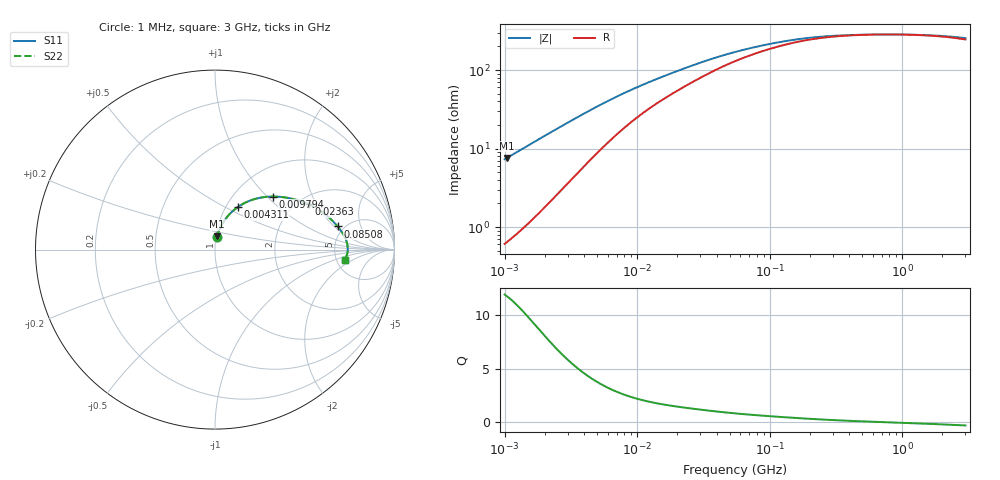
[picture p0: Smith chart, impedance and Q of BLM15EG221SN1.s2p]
! BLM15EG221SN1
# Hz S RI R 50
!Freq.(Hz) S11(Real) S11(Imag) S21(Real) S21(Imag) S12(Real) S12(Imag) S22(Real) S22(Imag)
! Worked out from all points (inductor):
!   401 points, 1 MHz to 3 GHz, reference 50 ohm
!   read as one part in series: L = 1.15 uH near 1.041 MHz
!   highest Q = 11.8 at 1.041 MHz (marker M1), where L = 1.16 uH
!   self-resonance near 825.3 MHz
!   S11 on the Smith chart (normalised r, x): 1 MHz: 1.01, +0.15; 4.311 MHz: 1.14, +0.59; 9.794 MHz: 1.49, +1.09; 23.63 MHz: 2.28, +1.73; 85.08 MHz: 4.41, +2.21; 3 GHz: 5.91, -1.39
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1000000  0.0112 0.0715  0.9888 -0.0715  0.9888 -0.0715  0.0112 0.0715
1040844  0.012 0.0743  0.988 -0.0743  0.988 -0.0743  0.012 0.0743
1553251  0.0235 0.1084  0.9765 -0.1084  0.9765 -0.1084  0.0235 0.1084
2182827  0.0426 0.1465  0.9574 -0.1465  0.9574 -0.1465  0.0426 0.1465
2947212  0.0712 0.1863  0.9288 -0.1863  0.9288 -0.1863  0.0712 0.1863
3823119  0.108 0.2225  0.892 -0.2225  0.892 -0.2225  0.108 0.2225
4310966  0.1293 0.2385  0.8707 -0.2385  0.8707 -0.2385  0.1293 0.2385
5266264  0.1704 0.2623  0.8296 -0.2623  0.8296 -0.2623  0.1704 0.2623
6433254  0.2175 0.2806  0.7825 -0.2806  0.7825 -0.2806  0.2175 0.2806
7858845  0.2681 0.2917  0.7319 -0.2917  0.7319 -0.2917  0.2681 0.2917
9794439  0.3247 0.2956  0.6753 -0.2956  0.6753 -0.2956  0.3247 0.2956
1.461624e7  0.422 0.2848  0.578 -0.2848  0.578 -0.2848  0.422 0.2848
2.362996e7  0.5232 0.2522  0.4768 -0.2522  0.4768 -0.2522  0.5232 0.2522
3.597591e7  0.594 0.2121  0.406 -0.2121  0.406 -0.2121  0.594 0.2121
5.477226e7  0.6456 0.1693  0.3544 -0.1693  0.3544 -0.1693  0.6456 0.1693
8.507507e7  0.6832 0.1291  0.3168 -0.1291  0.3168 -0.1291  0.6832 0.1291
1.348146e8  0.7104 0.0927  0.2896 -0.0927  0.2896 -0.0927  0.7104 0.0927
2.094008e8  0.7266 0.0628  0.2734 -0.0628  0.2734 -0.0628  0.7266 0.0628
3.817355e8  0.7369 0.0306  0.2631 -0.0306  0.2631 -0.0306  0.7369 0.0306
8.005644e8  0.7397 0.00111  0.2603 -0.00111  0.2603 -0.00111  0.7397 0.00111
1.645649e9  0.7356 -0.0268  0.2644 0.0268  0.2644 0.0268  0.7356 -0.0268
3e9  0.7218 -0.056  0.2782 0.056  0.2782 0.056  0.7218 -0.056
